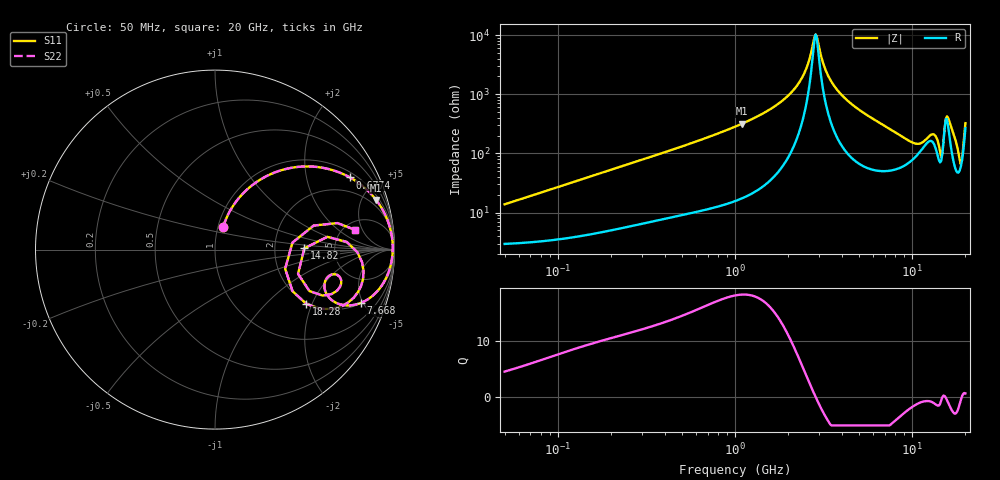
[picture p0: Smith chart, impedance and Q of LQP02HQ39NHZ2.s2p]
!Murata Part Number: LQP02HQ39NHZ2
!These Parameters are Measured in Series Mode Connection
!  o--[Z]--o
!Port1  Port2
!  o-------o
!Freq. Start=50[MHz] Stop=20[GHz], 401[Steps]
# Hz S RI R 50
!Freq.(Hz) S11(Real) S11(Imag) S21(Real) S21(Imag) S12(Real) S12(Imag) S22(Real) S22(Imag)
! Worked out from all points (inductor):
!   401 points, 50 MHz to 20 GHz, reference 50 ohm
!   read as one part in series: L = 42.9 nH near 51.52 MHz
!   highest Q = 18.2 at 1.094 GHz (marker M1), where L = 46.2 nH
!   self-resonance near 2.853 GHz
!   S11 on the Smith chart (normalised r, x): 50 MHz: 1.06, +0.27; 677.4 MHz: 1.22, +3.60; 7.668 GHz: 2.04, -4.84; 14.82 GHz: 2.98, +0.06; 18.28 GHz: 1.95, -1.82; 20 GHz: 6.35, +3.69
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5e7  0.0452 0.1253  0.9548 -0.1253  0.9548 -0.1253  0.0452 0.1253
1.364002e8  0.1435 0.2994  0.8565 -0.2994  0.8565 -0.2994  0.1435 0.2994
3.721004e8  0.4875 0.4628  0.5125 -0.4628  0.5125 -0.4628  0.4875 0.4628
6.774326e8  0.7517 0.4022  0.2483 -0.4022  0.2483 -0.4022  0.7517 0.4022
1e9  0.876 0.3031  0.124 -0.3031  0.124 -0.3031  0.876 0.3031
1.094034e9  0.8974 0.2772  0.1026 -0.2772  0.1026 -0.2772  0.8974 0.2772
2.083303e9  0.9826 0.0897  0.0174 -0.0897  0.0174 -0.0897  0.9826 0.0897
2.456456e9  0.989 0.0429  0.011 -0.0429  0.011 -0.0429  0.989 0.0429
2.728004e9  0.9904 0.0133  0.0096 -0.0133  0.0096 -0.0133  0.9904 0.0133
2.896447e9  0.9902 -0.00375  0.00976 0.00375  0.00976 0.00375  0.9902 -0.00375
3.314454e9  0.9872 -0.0424  0.0128 0.0424  0.0128 0.0424  0.9872 -0.0424
4.026975e9  0.9756 -0.0998  0.0244 0.0998  0.0244 0.0998  0.9756 -0.0998
7.442007e9  0.8296 -0.2895  0.1704 0.2895  0.1704 0.2895  0.8296 -0.2895
7.668323e9  0.8143 -0.2965  0.1857 0.2965  0.1857 0.2965  0.8143 -0.2965
1.004137e10  0.6369 -0.2686  0.3631 0.2686  0.3631 0.2686  0.6369 -0.2686
1.220001e10  0.6585 -0.1374  0.3415 0.1374  0.3415 0.1374  0.6585 -0.1374
1.396067e10  0.6507 -0.2474  0.3493 0.2474  0.3493 0.2474  0.6507 -0.2474
1.482269e10  0.4978 0.00714  0.5022 -0.00714  0.5022 -0.00714  0.4978 0.00714
1.597544e10  0.8274 -0.1194  0.1726 0.1194  0.1726 0.1194  0.8274 -0.1194
1.828096e10  0.5091 -0.303  0.4909 0.303  0.4909 0.303  0.5091 -0.303
1.88369e10  0.3908 -0.1065  0.6092 0.1065  0.6092 0.1065  0.3908 -0.1065
2e10  0.7827 0.1092  0.2173 -0.1092  0.2173 -0.1092  0.7827 0.1092
